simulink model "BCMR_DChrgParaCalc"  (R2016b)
settings: Solver=FixedStepDiscrete  StartTime=0.0  StopTime=10  FixedStep=0.01  RelTol=1e-3  EnableMultiTasking=on
undefined symbols (not defined in the file or in its folder): BCMR_ahDChgBattNominalCapa_C, BCMR_bCurrCalSelect_C, BCMR_bCurrIncDeltaLimEna_C, BCMR_bDChrgFulChkTenEna_C, BCMR_bDChrgFulChkThreeEna_C, BCMR_cntCoolDFC_CW, BCMR_cntSoh_CW, BCMR_G1E0PlatformSwPara_C, BCMR_iCurrDcr_C, BCMR_iDcChrgCurrAbnorm_T, BCMR_iDcChrgCurrAbnormMAP_T, BCMR_iDcChrgCurrNew_T, BCMR_iDcChrgCurrNewMAP_T, BCMR_iDcChrgCurrOld_T, BCMR_iDcChrgCurrOldAbnorm_T, BCMR_iDcChrgCurrOldAbnormMAP_T, BCMR_iDcChrgCurrOldMAP_T, BCMR_iDCCurrDecStep_C, BCMR_iDCCurrDecThrd_C, BCMR_iDCCurrDeltaLim_C, BCMR_iDCCurrDiff_C, BCMR_iDCCurrFil_C, BCMR_iDCCurrIncStep_C, BCMR_iDCCurrIncThrd_C, BCMR_iDChrgCurrCutOff_C, BCMR_kmAcmDist_C, BCMR_numCcsPwrSelc_C, BCMR_numCellVoltFull_C, BCMR_numCellVoltFullThree_C, BCMR_numCurrCalcEna, BCMR_pCcsPwrSelc_C, BCMR_pctBmsPwrRdc_C, BCMR_rCurrDcr_C, BCMR_rCurrIcr_C, BCMR_rDchrgLoadCoef_C, BCMR_tBattTempMaxFil_C, BCMR_tBattTempSelcLmtDwn_C, BCMR_tBattTempSelcLmtUp_C, BCMR_tDcChrgCellTemp1_A, BCMR_tDcChrgCellTemp2_A, BCMR_tDcChrgCellTemp_A, BCMR_tDchrgLoadLmt_C, BCMR_tiBattTempMaxFilDly_C, BCMR_tiBattTempSwitch_C, BCMR_tiCellVoltFullCnt_C, BCMR_tiCellVoltMaxFilDly_C, BCMR_tiCurrHysTimeDelay_C, BCMR_tiDcChrgPwrCCSDebs_C, BCMR_tiDChgFullPreHold_C, BCMR_tiDChrgCurrReqCalDly_C, BCMR_tiDChrgDetParaDebs_C, BCMR_tiDChrgFullBase_C, BCMR_tiDChrgFullDebs_C, BCMR_tiDChrgFulParaDebs_C, BCMR_tiDChrgFulWait_C, BCMR_tiDChrgParaBase_C, BCMR_tiHoldOnToCurrCalcOff_C, BCMR_tTempDisMapX_A, BCMR_tTempDisMapY_A, BCMR_uBattVoltOff_C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
libraries: simulink x34
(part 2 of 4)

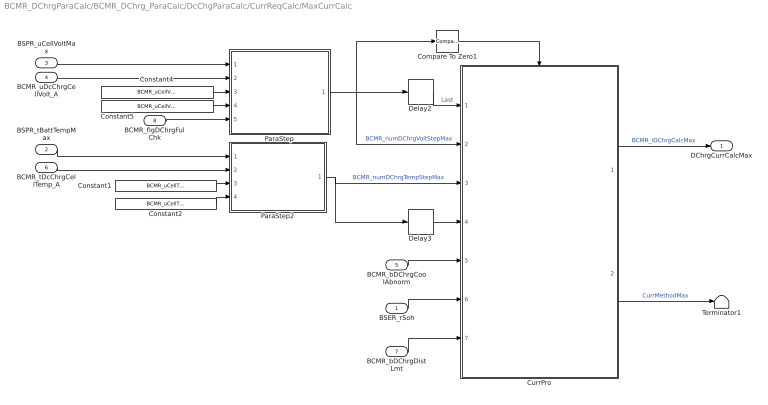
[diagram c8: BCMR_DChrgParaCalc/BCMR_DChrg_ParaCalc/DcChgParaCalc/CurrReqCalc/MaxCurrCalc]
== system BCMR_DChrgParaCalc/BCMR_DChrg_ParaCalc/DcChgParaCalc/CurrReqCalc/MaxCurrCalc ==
  BSER_rSoh : Inport
  BSPR_tBattTempMax : Inport  Port=2
  BSPR_uCellVoltMax : Inport  Port=3
  BCMR_uDcChrgCellVolt_A : Inport  Port=4
  BCMR_bDChrgCoolAbnorm : Inport  Port=5
  BCMR_tDcChrgCellTemp_A : Inport  Port=6
  BCMR_bDChrgDistLmt : Inport  Port=7
  BCMR_flgDChrgFulChk : Inport  Port=8
  Compare To Zero1 : simulink/Logic and Bit Operations/Compare To Zero  relop=>=  OutDataTypeStr=boolean
  Constant1 : Constant  Value=BCMR_uCellTempStep_A
  Constant2 : Constant  Value=BCMR_uCellTempHysRng_C
  Constant4 : Constant  Value=BCMR_uCellVoltStep_A
  Constant5 : Constant  Value=BCMR_uCellVoltHysRng_C
  CurrPro : Subsystem
  Delay2 : Delay  DelayLength=1  InitialCondition=0
  Delay3 : Delay  DelayLength=1  InitialCondition=0
  ParaStep : Stateflow chart  TreatAsAtomicUnit=on
  ParaStep2 : Stateflow chart  TreatAsAtomicUnit=on
  Terminator1 : Terminator
  DChrgCurrCalcMax : Outport
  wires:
  CurrPro/1(CurrCalc) -> DChrgCurrCalcMax/1  "BCMR_iDChrgCalcMax"
  ParaStep/1(ParaStep) -> Compare To Zero1/1, CurrPro/2(VoltStepN), Delay2/1  "BCMR_numDChrgVoltStepMax"
  Constant2/1 -> ParaStep2/4(BCMR_HysRng_C)
  ParaStep2/1(ParaStep) -> CurrPro/3(TempStepN), Delay3/1  "BCMR_numDChrgTempStepMax"
  BSPR_uCellVoltMax/1 -> ParaStep/1(BattTemp)
  BCMR_tDcChrgCellTemp_A/1 -> ParaStep2/2(BCMR_BattPara_A)
  Compare To Zero1/1 -> CurrPro/Enable
  Delay2/1 -> CurrPro/1(VoltStepL)  "Last"
  Constant1/1 -> ParaStep2/3(BCMR_ParaStep_A)
  Delay3/1 -> CurrPro/4(TempStepL)
  BCMR_uDcChrgCellVolt_A/1 -> ParaStep/2(BCMR_BattPara_A)
  BSPR_tBattTempMax/1 -> ParaStep2/1(BattTemp)
  CurrPro/2(CurrMethod) -> Terminator1/1  "CurrMethodMax"
  Constant5/1 -> ParaStep/4(BCMR_HysRng_C)
  Constant4/1 -> ParaStep/3(BCMR_ParaStep_A)
  BCMR_flgDChrgFulChk/1 -> ParaStep/5(BCMR_flgDChrgFulChk)
  BCMR_bDChrgCoolAbnorm/1 -> CurrPro/5(BCMR_bDChrgCoolAbnorm)
  BSER_rSoh/1 -> CurrPro/6(BSER_rSoh)
  BCMR_bDChrgDistLmt/1 -> CurrPro/7(BCMR_bDChrgDistLmt)

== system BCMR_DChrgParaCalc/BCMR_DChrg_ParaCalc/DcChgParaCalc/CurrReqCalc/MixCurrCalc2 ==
  BSER_rSoh : Inport
  BSPR_tBattTempMax : Inport  Port=2
  BSPR_uCellVoltMax : Inport  Port=3
  BCMR_uDcChrgCellVolt_A : Inport  Port=4
  BCMR_bDChrgCoolAbnorm : Inport  Port=5
  BCMR_tDcChrgCellTemp_A : Inport  Port=6
  BCMR_bDChrgDistLmt : Inport  Port=7
  BCMR_flgDChrgFulChk : Inport  Port=8
  Compare To Zero1 : simulink/Logic and Bit Operations/Compare To Zero  relop=>=  OutDataTypeStr=boolean
  Constant1 : Constant  Value=BCMR_uCellTempStep_A
  Constant2 : Constant  Value=BCMR_uCellTempHysRng_C
  Constant7 : Constant  Value=BCMR_uCellVoltStep_A
  Constant8 : Constant  Value=BCMR_uCellVoltHysRng_C
  CurrPro : Subsystem
  Delay2 : Delay  DelayLength=1  InitialCondition=0
  Delay3 : Delay  DelayLength=1  InitialCondition=0
  ParaStep : Stateflow chart  TreatAsAtomicUnit=on
  ParaStep1 : Stateflow chart  TreatAsAtomicUnit=on
  Terminator1 : Terminator
  DChrgCurrCalcMix2 : Outport
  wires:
  CurrPro/1(CurrCalc) -> DChrgCurrCalcMix2/1  "BCMR_iDChrgCalcMix2"
  ParaStep/1(ParaStep) -> CurrPro/2(VoltStepN), Delay2/1, Compare To Zero1/1  "BCMR_numDChrgVoltStepMix2"
  Constant2/1 -> ParaStep1/4(BCMR_HysRng_C)
  ParaStep1/1(ParaStep) -> CurrPro/3(TempStepN), Delay3/1  "BCMR_numDChrgTempStepMix2"
  BCMR_tDcChrgCellTemp_A/1 -> ParaStep1/2(BCMR_BattPara_A)
  Compare To Zero1/1 -> CurrPro/Enable
  Delay2/1 -> CurrPro/1(VoltStepL)  "Last"
  Constant1/1 -> ParaStep1/3(BCMR_ParaStep_A)
  Delay3/1 -> CurrPro/4(TempStepL)
  CurrPro/2(CurrMethod) -> Terminator1/1  "CurrMethodMin"
  BSPR_uCellVoltMax/1 -> ParaStep/1(BattTemp)
  BCMR_uDcChrgCellVolt_A/1 -> ParaStep/2(BCMR_BattPara_A)
  Constant8/1 -> ParaStep/4(BCMR_HysRng_C)
  Constant7/1 -> ParaStep/3(BCMR_ParaStep_A)
  BCMR_flgDChrgFulChk/1 -> ParaStep/5(BCMR_flgDChrgFulChk)
  BCMR_bDChrgCoolAbnorm/1 -> CurrPro/5(BCMR_bDChrgCoolAbnorm)
  BSER_rSoh/1 -> CurrPro/6(BSER_rSoh)
  BSPR_tBattTempMax/1 -> ParaStep1/1(BattTemp)
  BCMR_bDChrgDistLmt/1 -> CurrPro/7(BCMR_bDChrgDistLmt)

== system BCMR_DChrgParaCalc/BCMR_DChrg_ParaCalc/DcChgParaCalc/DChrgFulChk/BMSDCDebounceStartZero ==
  Signal : Inport
  Hearl2Fault : Inport  Port=2
  FaultStep : Inport  Port=3
  Fault2Heal : Inport  Port=4
  HealStep : Inport  Port=5
  Compare To Zero : simulink/Logic and Bit Operations/Compare To Zero  relop===  OutDataTypeStr=boolean
  FaultProcess : Subsystem
  HealProcess : Subsystem
  Switch : Switch  Criteria=u2 ~= 0
  Unit Delay : UnitDelay  SampleTime=-1  StateName=StateName
  FaultFlag : Outport  OutDataTypeStr=boolean
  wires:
  Compare To Zero/1 -> Switch/2
  Unit Delay/1 -> Compare To Zero/1, FaultProcess/4(FaultFlagOldState), HealProcess/4(FaultFlagOldState)
  HealStep/1 -> HealProcess/3(HealStep)
  Fault2Heal/1 -> HealProcess/2(Fault2Heal)
  Signal/1 -> FaultProcess/1(Signal), HealProcess/1(Signal)
  FaultStep/1 -> FaultProcess/3(FaultStep)
  Hearl2Fault/1 -> FaultProcess/2(Hearl2Fault)
  Switch/1 -> Unit Delay/1, FaultFlag/1
  HealProcess/1(FaultFlag) -> Switch/3
  FaultProcess/1(FaultFlag) -> Switch/1

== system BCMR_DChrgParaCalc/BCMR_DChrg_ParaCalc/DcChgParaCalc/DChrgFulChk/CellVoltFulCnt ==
  En : Inport
  Rst : Inport  Port=2
  Compare To Constant : simulink/Logic and Bit Operations/Compare To Constant  relop=>=  const=BCMR_numCellVoltFull_C  OutDataTypeStr=boolean
  Compare To Constant1 : simulink/Logic and Bit Operations/Compare To Constant  relop=>=  const=BCMR_numCellVoltFullThree_C  OutDataTypeStr=boolean
  Constant1 : Constant  Value=0  OutDataTypeStr=uint8
  Constant2 : Constant  OutDataTypeStr=uint8
  EdgeRising : Subsystem  TreatAsAtomicUnit=on  RTWFcnName=EdgeRising  RTWFileName=SrvLib
  EdgeRising1 : Subsystem  TreatAsAtomicUnit=on  RTWFcnName=EdgeRising  RTWFileName=SrvLib
  Timer : Subsystem
  Ten : Outport
  Three : Outport  Port=2
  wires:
  Compare To Constant/1 -> Ten/1  "BCMR_bCellVoltFullCnt"
  EdgeRising/1(y) -> Timer/1(En)
  Constant1/1 -> Timer/4(Vst)
  EdgeRising1/1(y) -> Timer/3(Rst)
  En/1 -> EdgeRising/1(u)
  Constant2/1 -> Timer/2(Cnt)
  Timer/1(Number) -> Compare To Constant1/1, Compare To Constant/1  "BCMR_numCellVoltFullCnt"
  Rst/1 -> EdgeRising1/1(u)
  Compare To Constant1/1 -> Three/1  "BCMR_bCellVoltFullTriger"

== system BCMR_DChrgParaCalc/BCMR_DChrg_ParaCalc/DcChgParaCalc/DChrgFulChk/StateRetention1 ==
  u : Inport
  clc : Inport  Port=2
  Constant1 : Constant  Value=BCMR_tiDChrgParaBase_C
  Constant2 : Constant  Value=BCMR_tiCellVoltFullCnt_C
  Constant8 : Constant  Value=single(0)
  Delay2 : Delay  DelayLength=1  InitialCondition=0
  EdgeRising : Subsystem  TreatAsAtomicUnit=on  RTWFcnName=EdgeRising  RTWFileName=SrvLib
  Logical Operator : Logic  Operator=OR  AllPortsSameDT=off  OutDataTypeStr=boolean
  Relational Operator2 : RelationalOperator  Operator=>  OutDataTypeStr=boolean  RndMeth=Simplest
  Subsystem3 : Subsystem
  Timer : Subsystem
  BCMR_bCellVoltFullTmr : Outport
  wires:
  Subsystem3/1(Q) -> Timer/1(En)  "BCMR_bCellVoltFullTmrRaw"
  Delay2/1 -> EdgeRising/1(u), Logical Operator/2
  Constant2/1 -> Relational Operator2/2
  Constant8/1 -> Timer/4(Vst)
  Timer/1(Timer) -> Relational Operator2/1
  EdgeRising/1(y) -> Timer/3(Rst)
  Constant1/1 -> Timer/2(Ts)
  Relational Operator2/1 -> BCMR_bCellVoltFullTmr/1, Delay2/1  "BCMR_bCellVoltFullTmr"
  u/1 -> Subsystem3/1(set)
  Logical Operator/1 -> Subsystem3/2(clear)
  clc/1 -> Logical Operator/1

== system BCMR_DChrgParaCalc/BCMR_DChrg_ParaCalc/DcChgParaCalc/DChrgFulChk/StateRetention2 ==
  u : Inport
  Constant4 : Constant  Value=BCMR_tiDChrgParaBase_C
  Constant5 : Constant  Value=BCMR_tiDChgFullPreHold_C
  Constant8 : Constant  Value=single(0)
  Delay2 : Delay  DelayLength=1  InitialCondition=0
  EdgeRising : Subsystem  TreatAsAtomicUnit=on  RTWFcnName=EdgeRising  RTWFileName=SrvLib
  Relational Operator2 : RelationalOperator  Operator=>  OutDataTypeStr=boolean  RndMeth=Simplest
  Subsystem3 : Subsystem
  Timer : Subsystem
  BCMR_flgDChrgFulChk : Outport
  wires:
  Subsystem3/1(Q) -> BCMR_flgDChrgFulChk/1, Timer/1(En)  "BCMR_flgDChrgFulChk"
  Delay2/1 -> EdgeRising/1(u), Subsystem3/2(clear)
  Constant5/1 -> Relational Operator2/2
  Constant8/1 -> Timer/4(Vst)
  Timer/1(Timer) -> Relational Operator2/1
  EdgeRising/1(y) -> Timer/3(Rst)
  Constant4/1 -> Timer/2(Ts)
  Relational Operator2/1 -> Delay2/1
  u/1 -> Subsystem3/1(set)  "BCMR_flgDChrgFulChkRaw"

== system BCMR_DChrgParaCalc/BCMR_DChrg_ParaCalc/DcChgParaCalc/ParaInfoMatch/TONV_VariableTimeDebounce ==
  note: Turn On Delay Time Deboune
  u : Inport
  T : Inport  Port=2
  dT : Inport  Port=3
  Add : Sum
  Constant1 : Constant  Value=0  OutDataTypeStr=single
  Constant2 : Constant  OutDataTypeStr=uint8
  Constant3 : Constant  Value=0  OutDataTypeStr=uint8
  Delay : Delay  DelayLength=1  InitialCondition=0
  MinMax : MinMax  Inputs=2
  Product : Product  OutMin=[0]  OutMax=[65535]  OutDataTypeStr=single
  Relational Operator : RelationalOperator  Operator=>  OutDataTypeStr=boolean  RndMeth=Simplest
  Switch : Switch  Criteria=u2 ~= 0
  Switch1 : Switch  Criteria=u2 ~= 0
  y : Outport
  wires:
  Switch1/1 -> Product/1
  Constant3/1 -> Switch1/3
  Constant2/1 -> Switch1/1
  u/1 -> Switch1/2, Switch/2
  dT/1 -> Switch/1
  Constant1/1 -> Switch/3
  Add/1 -> Product/2
  Product/1 -> Relational Operator/1, Delay/1
  Switch/1 -> Add/1
  Delay/1 -> MinMax/2
  Relational Operator/1 -> y/1
  T/1 -> MinMax/1, Relational Operator/2
  MinMax/1 -> Add/2

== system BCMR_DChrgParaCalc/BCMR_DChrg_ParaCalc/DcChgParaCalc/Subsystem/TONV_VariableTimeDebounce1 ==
  note: Turn On Delay Time Deboune
  u : Inport
  T : Inport  Port=2
  dT : Inport  Port=3
  Add : Sum
  Constant1 : Constant  Value=0  OutDataTypeStr=single
  Constant2 : Constant  OutDataTypeStr=uint8
  Constant3 : Constant  Value=0  OutDataTypeStr=uint8
  Delay : Delay  DelayLength=1  InitialCondition=0
  MinMax : MinMax  Inputs=2
  Product : Product  OutMin=[0]  OutMax=[65535]  OutDataTypeStr=single
  Relational Operator : RelationalOperator  Operator=>  OutDataTypeStr=boolean  RndMeth=Simplest
  Switch : Switch  Criteria=u2 ~= 0
  Switch1 : Switch  Criteria=u2 ~= 0
  y : Outport
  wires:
  Switch1/1 -> Product/1
  Constant3/1 -> Switch1/3
  Constant2/1 -> Switch1/1
  u/1 -> Switch1/2, Switch/2
  dT/1 -> Switch/1
  Constant1/1 -> Switch/3
  Add/1 -> Product/2
  Product/1 -> Relational Operator/1, Delay/1
  Switch/1 -> Add/1
  Delay/1 -> MinMax/2
  Relational Operator/1 -> y/1
  T/1 -> MinMax/1, Relational Operator/2
  MinMax/1 -> Add/2

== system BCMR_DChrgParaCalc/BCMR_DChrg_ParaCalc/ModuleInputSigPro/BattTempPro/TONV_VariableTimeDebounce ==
  note: Turn On Delay Time Deboune
  u : Inport
  T : Inport  Port=2
  dT : Inport  Port=3
  Add : Sum
  Constant1 : Constant  Value=0  OutDataTypeStr=single
  Constant2 : Constant  OutDataTypeStr=uint8
  Constant3 : Constant  Value=0  OutDataTypeStr=uint8
  Delay : Delay  DelayLength=1  InitialCondition=0
  MinMax : MinMax  Inputs=2
  Product : Product  OutMin=[0]  OutMax=[65535]  OutDataTypeStr=single
  Relational Operator : RelationalOperator  Operator=>  OutDataTypeStr=boolean  RndMeth=Simplest
  Switch : Switch  Criteria=u2 ~= 0
  Switch1 : Switch  Criteria=u2 ~= 0
  y : Outport
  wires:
  Switch1/1 -> Product/1
  Constant3/1 -> Switch1/3
  Constant2/1 -> Switch1/1
  u/1 -> Switch1/2, Switch/2
  dT/1 -> Switch/1
  Constant1/1 -> Switch/3
  Add/1 -> Product/2
  Product/1 -> Relational Operator/1, Delay/1
  Switch/1 -> Add/1
  Delay/1 -> MinMax/2
  Relational Operator/1 -> y/1
  T/1 -> MinMax/1, Relational Operator/2
  MinMax/1 -> Add/2

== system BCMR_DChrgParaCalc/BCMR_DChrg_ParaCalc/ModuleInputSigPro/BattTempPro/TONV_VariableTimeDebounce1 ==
  note: Turn On Delay Time Deboune
  u : Inport
  T : Inport  Port=2
  dT : Inport  Port=3
  Add : Sum
  Constant1 : Constant  Value=0  OutDataTypeStr=single
  Constant2 : Constant  OutDataTypeStr=uint8
  Constant3 : Constant  Value=0  OutDataTypeStr=uint8
  Delay : Delay  DelayLength=1  InitialCondition=0
  MinMax : MinMax  Inputs=2
  Product : Product  OutMin=[0]  OutMax=[65535]  OutDataTypeStr=single
  Relational Operator : RelationalOperator  Operator=>  OutDataTypeStr=boolean  RndMeth=Simplest
  Switch : Switch  Criteria=u2 ~= 0
  Switch1 : Switch  Criteria=u2 ~= 0
  y : Outport
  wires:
  Switch1/1 -> Product/1
  Constant3/1 -> Switch1/3
  Constant2/1 -> Switch1/1
  u/1 -> Switch1/2, Switch/2
  dT/1 -> Switch/1
  Constant1/1 -> Switch/3
  Add/1 -> Product/2
  Product/1 -> Relational Operator/1, Delay/1
  Switch/1 -> Add/1
  Delay/1 -> MinMax/2
  Relational Operator/1 -> y/1
  T/1 -> MinMax/1, Relational Operator/2
  MinMax/1 -> Add/2

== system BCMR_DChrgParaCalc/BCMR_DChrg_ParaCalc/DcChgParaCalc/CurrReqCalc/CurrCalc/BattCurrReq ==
  Curr : Inport
  BCMR_flgDChrgPwrRdc : Inport  Port=2
  CurrPro : Subsystem
  BCMR_iDChrgBattCurrReqCalc : Outport  OutputWhenDisabled=reset  InitialOutput=[0]
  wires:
  BCMR_flgDChrgPwrRdc/1 -> CurrPro/2(BCMR_flgDChrgPwrRdc)
  CurrPro/1(BCMR_iDChrgBattCurrReqCalc) -> BCMR_iDChrgBattCurrReqCalc/1
  Curr/1 -> CurrPro/1(CurrPro)

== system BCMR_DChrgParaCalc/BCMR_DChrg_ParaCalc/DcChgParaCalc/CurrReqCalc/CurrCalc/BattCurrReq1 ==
  CurrReq : Inport
  COMR_iDcChrgMaxCurrOutputPmtdCml : Inport  Port=2
  COMR_tiDcChrgTimeActualCcs : Inport  Port=3
  COMR_iDcChrgOutputCurrCcs : Inport  Port=4
  COMR_iDcChrgMinCurrOutputPmtdCml : Inport  Port=5
  BSPR_uPackVolt : Inport  Port=6
  BCMR_stDChrgMode : Inport  Port=7
  CurrPro : Subsystem
  BCMR_iDChrgBattCurrReqCalc : Outport  OutputWhenDisabled=reset  InitialOutput=[0]
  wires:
  COMR_iDcChrgMaxCurrOutputPmtdCml/1 -> CurrPro/2(COMR_iDcChrgMaxCurrOutputPmtdCml)
  CurrPro/1(BCMR_iDChrgBattCurrReqCalc) -> BCMR_iDChrgBattCurrReqCalc/1
  CurrReq/1 -> CurrPro/1(CurrReq)
  COMR_tiDcChrgTimeActualCcs/1 -> CurrPro/4(COMR_tiDcChrgTimeActualCcs)
  COMR_iDcChrgOutputCurrCcs/1 -> CurrPro/5(COMR_iDcChrgOutputCurrCcs)
  COMR_iDcChrgMinCurrOutputPmtdCml/1 -> CurrPro/3(COMR_iDcChrgMinCurrOutputPmtdCml)
  BSPR_uPackVolt/1 -> CurrPro/6(BSPR_uPackVolt)
  BCMR_stDChrgMode/1 -> CurrPro/7(BCMR_stDChrgMode)

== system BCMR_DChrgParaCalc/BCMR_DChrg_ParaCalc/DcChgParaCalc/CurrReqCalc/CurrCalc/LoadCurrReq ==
  COMR_pwrChrgLdReq : Inport
  BSPR_uPackVolt : Inport  Port=2
  BSPR_tBattTempMin : Inport  Port=3
  Compare To Constant : simulink/Logic and Bit Operations/Compare To Constant  relop=>=  const=BCMR_tDchrgLoadLmt_C  OutDataTypeStr=boolean
  Constant : Constant  Value=408  OutDataTypeStr=single
  Constant2 : Constant  Value=0  OutDataTypeStr=single
  Divide : Product  Inputs=*/
  Gain : Gain  Gain=1000
  Gain1 : Gain  Gain=BCMR_rDchrgLoadCoef_C
  SIgFil1 : Subsystem
  Switch : Switch  Criteria=u2 > Threshold
  Switch1 : Switch  Criteria=u2 > Threshold
  BCMR_iDChrgLoadCurrReqCalc : Outport
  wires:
  COMR_pwrChrgLdReq/1 -> Gain/1
  BSPR_uPackVolt/1 -> Switch/1, Switch/2
  Switch/1 -> Divide/2
  Constant/1 -> Switch/3
  Divide/1 -> Gain1/1
  Gain1/1 -> BCMR_iDChrgLoadCurrReqCalc/1
  BSPR_tBattTempMin/1 -> Compare To Constant/1
  Compare To Constant/1 -> Switch1/2
  Gain/1 -> [COMR_pwrChrgLdReq]
  [COMR_pwrChrgLdReq] -> SIgFil1/1(u)
  SIgFil1/1(y) -> Switch1/1
  Constant2/1 -> Switch1/3
  Switch1/1 -> Divide/1

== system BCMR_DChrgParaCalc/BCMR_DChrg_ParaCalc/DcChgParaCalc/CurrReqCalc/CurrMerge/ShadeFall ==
  In1 : Inport
  In2 : Inport  Port=2
  Add1 : Sum  Inputs=+-
  Constant3 : Constant  Value=BCMR_iCurrDcr_C  OutDataTypeStr=single
  MinMax1 : MinMax  Inputs=2
  MinMax2 : MinMax  Inputs=2
  MinMax3 : MinMax  Function=max  Inputs=2
  Relational Operator2 : RelationalOperator  OutDataTypeStr=boolean  RndMeth=Simplest
  Switch1 : Switch  Criteria=u2 > Threshold
  Unit Delay4 : UnitDelay  InitialCondition=1000  SampleTime=-1
  val : Outport
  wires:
  Constant3/1 -> Add1/2
  Add1/1 -> Switch1/1, Relational Operator2/1
  Relational Operator2/1 -> Switch1/2  "equalFlg"
  Switch1/1 -> Unit Delay4/1, val/1
  In1/1 -> MinMax1/1, MinMax3/1
  In2/1 -> MinMax1/2, MinMax3/2
  MinMax1/1 -> Switch1/3, Relational Operator2/2
  MinMax3/1 -> MinMax2/2
  Unit Delay4/1 -> MinMax2/1
  MinMax2/1 -> Add1/1

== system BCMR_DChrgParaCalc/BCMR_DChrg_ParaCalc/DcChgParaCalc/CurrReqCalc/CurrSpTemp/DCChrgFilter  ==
  In1 : Inport
  In2 : Inport  Port=2
  Abs : Abs
  Compare To Constant : simulink/Logic and Bit Operations/Compare To Constant  relop=>=  const=BCMR_iDCCurrDiff_C  OutDataTypeStr=boolean
  Subtract1 : Sum  Inputs=+-
  Switch2 : Switch  Criteria=u2 ~= 0
  Out1 : Outport
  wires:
  In2/1 -> Switch2/3, Subtract1/2
  Subtract1/1 -> Abs/1
  Abs/1 -> Compare To Constant/1
  Compare To Constant/1 -> Switch2/2
  Switch2/1 -> Out1/1
  In1/1 -> Subtract1/1, Switch2/1

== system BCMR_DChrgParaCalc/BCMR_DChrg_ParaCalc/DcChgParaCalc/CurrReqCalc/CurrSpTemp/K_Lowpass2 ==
  k : Inport
  u : Inport  Port=2
  Add : Sum
  Constant2 : Constant  Value=0
  Delay : Delay  DelayLength=1  InitialCondition=1
  Product : Product
  Subtract : Sum  Inputs=+-
  Switch1 : Switch  Criteria=u2 > Threshold
  Unit Delay : UnitDelay  SampleTime=-1
  y : Outport
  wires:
  k/1 -> Product/1
  Product/1 -> Add/1
  Constant2/1 -> Delay/1
  Unit Delay/1 -> Subtract/2, Add/2
  Subtract/1 -> Product/2
  Add/1 -> Switch1/3
  Delay/1 -> Switch1/2
  Switch1/1 -> y/1, Unit Delay/1
  u/1 -> Switch1/1, Subtract/1

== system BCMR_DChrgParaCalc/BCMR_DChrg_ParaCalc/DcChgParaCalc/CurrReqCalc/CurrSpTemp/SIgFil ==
  u : Inport
  Constant4 : Constant  Value=0  OutDataTypeStr=boolean
  Delay1 : Delay  DelayLength=1  InitialCondition=0
  Filter : Subsystem
  Switch4 : Switch  Criteria=u2 ~= 0
  Unit Delay1 : UnitDelay  InitialCondition=1  SampleTime=-1
  y : Outport
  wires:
  Delay1/1 -> Filter/2(In2)
  u/1 -> Filter/1(In1), Switch4/1
  Unit Delay1/1 -> Switch4/2
  Constant4/1 -> Unit Delay1/1
  Filter/1(Out1) -> Switch4/3
  Switch4/1 -> y/1, Delay1/1

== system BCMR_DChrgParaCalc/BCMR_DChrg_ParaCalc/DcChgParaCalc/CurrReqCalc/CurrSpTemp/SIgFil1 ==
  u : Inport
  Constant4 : Constant  Value=0  OutDataTypeStr=boolean
  Delay1 : Delay  DelayLength=1  InitialCondition=0
  Filter : Subsystem
  Switch4 : Switch  Criteria=u2 ~= 0
  Unit Delay1 : UnitDelay  InitialCondition=1  SampleTime=-1
  y : Outport
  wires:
  Switch4/1 -> Delay1/1, y/1
  Filter/1(Out1) -> Switch4/3
  Constant4/1 -> Unit Delay1/1
  Unit Delay1/1 -> Switch4/2
  u/1 -> Switch4/1, Filter/1(In1)
  Delay1/1 -> Filter/2(In2)

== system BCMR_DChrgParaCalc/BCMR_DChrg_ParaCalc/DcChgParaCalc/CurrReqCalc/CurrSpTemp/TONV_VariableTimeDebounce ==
  note: Turn On Delay Time Deboune
  u : Inport
  T : Inport  Port=2
  dT : Inport  Port=3
  Add : Sum
  Constant1 : Constant  Value=0  OutDataTypeStr=single
  Constant2 : Constant  OutDataTypeStr=uint8
  Constant3 : Constant  Value=0  OutDataTypeStr=uint8
  Delay : Delay  DelayLength=1  InitialCondition=0
  MinMax : MinMax  Inputs=2
  Product : Product  OutMin=[0]  OutMax=[65535]  OutDataTypeStr=single
  Relational Operator : RelationalOperator  Operator=>  OutDataTypeStr=boolean  RndMeth=Simplest
  Switch : Switch  Criteria=u2 ~= 0
  Switch1 : Switch  Criteria=u2 ~= 0
  y : Outport
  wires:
  Switch1/1 -> Product/1
  Constant3/1 -> Switch1/3
  Constant2/1 -> Switch1/1
  u/1 -> Switch1/2, Switch/2
  dT/1 -> Switch/1
  Constant1/1 -> Switch/3
  Add/1 -> Product/2
  Product/1 -> Relational Operator/1, Delay/1
  Switch/1 -> Add/1
  Delay/1 -> MinMax/2
  Relational Operator/1 -> y/1
  T/1 -> MinMax/1, Relational Operator/2
  MinMax/1 -> Add/2

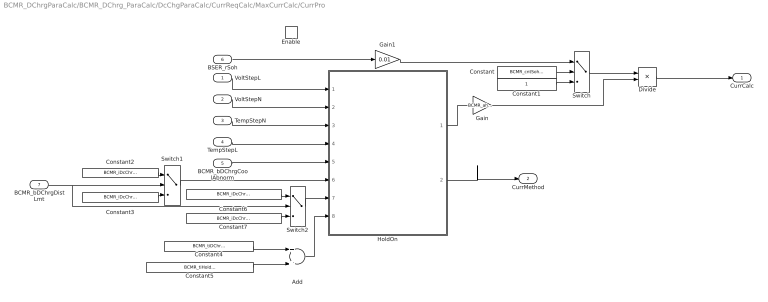
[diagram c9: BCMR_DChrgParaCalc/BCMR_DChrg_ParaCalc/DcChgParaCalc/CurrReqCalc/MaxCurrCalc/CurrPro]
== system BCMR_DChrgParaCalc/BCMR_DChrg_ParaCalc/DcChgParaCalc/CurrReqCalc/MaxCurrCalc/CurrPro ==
  VoltStepL : Inport
  VoltStepN : Inport  Port=2
  TempStepN : Inport  Port=3
  TempStepL : Inport  Port=4
  BCMR_bDChrgCoolAbnorm : Inport  Port=5
  BSER_rSoh : Inport  Port=6
  BCMR_bDChrgDistLmt : Inport  Port=7
  Enable : EnablePort  StatesWhenEnabling=reset
  Add : Sum
  Constant : Constant  Value=BCMR_cntSoh_CW
  Constant1 : Constant  OutDataTypeStr=single
  Constant2 : Constant  Value=BCMR_iDcChrgCurrOld_T
  Constant3 : Constant  Value=BCMR_iDcChrgCurrNew_T
  Constant4 : Constant  Value=BCMR_tiDChrgFulParaDebs_C
  Constant5 : Constant  Value=BCMR_tiHoldOnToCurrCalcOff_C
  Constant6 : Constant  Value=BCMR_iDcChrgCurrOldAbnorm_T
  Constant7 : Constant  Value=BCMR_iDcChrgCurrAbnorm_T
  Divide : Product  Inputs=**
  Gain : Gain  Gain=BCMR_ahDChgBattNominalCapa_C
  Gain1 : Gain  Gain=0.01  OutDataTypeStr=single
  HoldOn : Stateflow chart  TreatAsAtomicUnit=on
  Switch : Switch  Criteria=u2 > Threshold  Threshold=7
  Switch1 : Switch  Criteria=u2 > Threshold  Threshold=7
  Switch2 : Switch  Criteria=u2 > Threshold  Threshold=7
  CurrCalc : Outport  OutputWhenDisabled=reset  InitialOutput=[0]
  CurrMethod : Outport  Port=2  OutputWhenDisabled=reset  InitialOutput=[0]
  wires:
  HoldOn/1(CurrCalc) -> Gain/1
  VoltStepL/1 -> HoldOn/1(VoltStepLast)
  VoltStepN/1 -> HoldOn/2(VoltStepNext)
  TempStepN/1 -> HoldOn/3(TempStep)
  TempStepL/1 -> HoldOn/4(TempStepL)
  HoldOn/2(CurrMethod) -> CurrMethod/1
  Gain/1 -> Divide/2
  BCMR_bDChrgCoolAbnorm/1 -> HoldOn/5(BCMR_bDChrgCoolAbnorm)
  BSER_rSoh/1 -> Gain1/1
  Constant/1 -> Switch/2
  Constant1/1 -> Switch/3
  Gain1/1 -> Switch/1
  Switch/1 -> Divide/1
  Divide/1 -> CurrCalc/1
  Constant2/1 -> Switch1/1
  Constant3/1 -> Switch1/3
  Switch1/1 -> HoldOn/6(BCMR_iDcChrgCurrNew_T)
  BCMR_bDChrgDistLmt/1 -> Switch2/2, Switch1/2
  Constant6/1 -> Switch2/1
  Switch2/1 -> HoldOn/7(BCMR_iDcChrgCurrAbnorm_T)
  Constant7/1 -> Switch2/3
  Constant4/1 -> Add/1
  Constant5/1 -> Add/2
  Add/1 -> HoldOn/8(BCMR_tiHoldOnToCurrCalc_C)

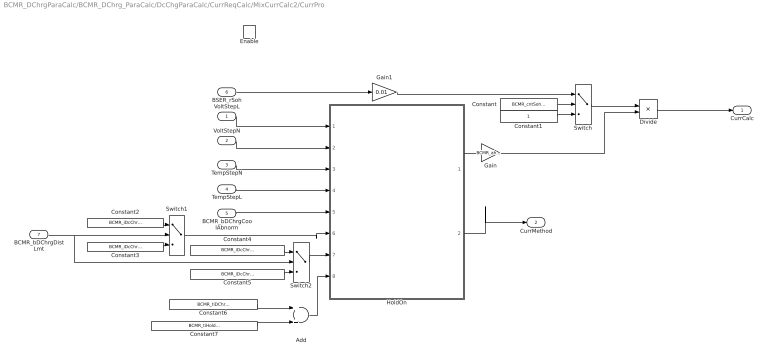
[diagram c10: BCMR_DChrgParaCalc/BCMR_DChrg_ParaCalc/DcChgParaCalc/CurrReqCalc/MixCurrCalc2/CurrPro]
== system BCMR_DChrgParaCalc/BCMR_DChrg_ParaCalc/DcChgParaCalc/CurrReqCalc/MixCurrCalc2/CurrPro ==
  VoltStepL : Inport
  VoltStepN : Inport  Port=2
  TempStepN : Inport  Port=3
  TempStepL : Inport  Port=4
  BCMR_bDChrgCoolAbnorm : Inport  Port=5
  BSER_rSoh : Inport  Port=6
  BCMR_bDChrgDistLmt : Inport  Port=7
  Enable : EnablePort  StatesWhenEnabling=reset
  Add : Sum
  Constant : Constant  Value=BCMR_cntSoh_CW
  Constant1 : Constant  OutDataTypeStr=single
  Constant2 : Constant  Value=BCMR_iDcChrgCurrOld_T
  Constant3 : Constant  Value=BCMR_iDcChrgCurrNew_T
  Constant4 : Constant  Value=BCMR_iDcChrgCurrOldAbnorm_T
  Constant5 : Constant  Value=BCMR_iDcChrgCurrAbnorm_T
  Constant6 : Constant  Value=BCMR_tiDChrgFulParaDebs_C
  Constant7 : Constant  Value=BCMR_tiHoldOnToCurrCalcOff_C
  Divide : Product  Inputs=**
  Gain : Gain  Gain=BCMR_ahDChgBattNominalCapa_C
  Gain1 : Gain  Gain=0.01  OutDataTypeStr=single
  HoldOn : Stateflow chart  TreatAsAtomicUnit=on
  Switch : Switch  Criteria=u2 > Threshold  Threshold=7
  Switch1 : Switch  Criteria=u2 > Threshold  Threshold=7
  Switch2 : Switch  Criteria=u2 > Threshold  Threshold=7
  CurrCalc : Outport  OutputWhenDisabled=reset  InitialOutput=[0]
  CurrMethod : Outport  Port=2  OutputWhenDisabled=reset  InitialOutput=[0]
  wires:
  HoldOn/1(CurrCalc) -> Gain/1
  VoltStepL/1 -> HoldOn/1(VoltStepLast)
  VoltStepN/1 -> HoldOn/2(VoltStepNext)
  TempStepN/1 -> HoldOn/3(TempStep)
  TempStepL/1 -> HoldOn/4(TempStepL)
  HoldOn/2(CurrMethod) -> CurrMethod/1
  Gain/1 -> Divide/2
  BCMR_bDChrgCoolAbnorm/1 -> HoldOn/5(BCMR_bDChrgCoolAbnorm)
  BSER_rSoh/1 -> Gain1/1
  Constant/1 -> Switch/2
  Constant1/1 -> Switch/3
  Gain1/1 -> Switch/1
  Switch/1 -> Divide/1
  Divide/1 -> CurrCalc/1
  Constant2/1 -> Switch1/1
  Constant3/1 -> Switch1/3
  Switch1/1 -> HoldOn/6(BCMR_iDcChrgCurrNew_T)
  BCMR_bDChrgDistLmt/1 -> Switch2/2, Switch1/2
  Constant4/1 -> Switch2/1
  Constant5/1 -> Switch2/3
  Switch2/1 -> HoldOn/7(BCMR_iDcChrgCurrAbnorm_T)
  Constant6/1 -> Add/1
  Add/1 -> HoldOn/8(BCMR_tiHoldOnToCurrCalc_C)
  Constant7/1 -> Add/2

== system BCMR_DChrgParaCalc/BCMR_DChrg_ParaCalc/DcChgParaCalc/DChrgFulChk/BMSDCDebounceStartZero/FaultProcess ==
  Signal : Inport
  Hearl2Fault : Inport  Port=2
  FaultStep : Inport  Port=3
  FaultFlagOldState : Inport  Port=4
  Constant : Constant  OutDataTypeStr=Inherit: Inherit via back propagation
  Constant1 : Constant  Value=0  OutDataTypeStr=Inherit: Inherit via back propagation
  Decrease : Subsystem
  Increase : Subsystem
  Relational Operator : RelationalOperator  Operator=>  OutDataTypeStr=boolean
  Switch : Switch  Criteria=u2 ~= 0
  Switch1 : Switch  Criteria=u2 ~= 0
  Switch2 : Switch  Criteria=u2 ~= 0
  Unit Delay : UnitDelay  SampleTime=-1  StateName=StateName
  Unit Delay1 : UnitDelay  SampleTime=-1  StateName=StateName
  FaultFlag : Outport
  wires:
  Unit Delay1/1 -> Switch2/2
  Unit Delay/1 -> Switch2/3
  Switch2/1 -> Increase/2(Counter), Decrease/2(Counter)
  Constant1/1 -> Switch2/1
  Constant/1 -> Switch/1
  FaultFlagOldState/1 -> Switch/3
  Switch/1 -> FaultFlag/1
  Relational Operator/1 -> Switch/2, Unit Delay1/1
  FaultStep/1 -> Increase/1(FaultStep), Decrease/1(FaultStep)
  Hearl2Fault/1 -> Relational Operator/2
  Switch1/1 -> Relational Operator/1, Unit Delay/1
  Decrease/1(FaultCnt) -> Switch1/3
  Increase/1(FaultCnt) -> Switch1/1
  Signal/1 -> Switch1/2

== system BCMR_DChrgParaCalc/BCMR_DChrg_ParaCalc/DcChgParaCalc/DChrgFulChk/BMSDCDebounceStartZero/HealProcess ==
  Signal : Inport
  Fault2Heal : Inport  Port=2
  HealStep : Inport  Port=3
  FaultFlagOldState : Inport  Port=4
  Compare To Zero : simulink/Logic and Bit Operations/Compare To Zero  relop===  OutDataTypeStr=boolean
  Constant : Constant  Value=0  OutDataTypeStr=Inherit: Inherit via back propagation
  Constant1 : Constant  Value=0  OutDataTypeStr=Inherit: Inherit via back propagation
  Decrease : Subsystem
  Increase : Subsystem
  Relational Operator : RelationalOperator  Operator=>  OutDataTypeStr=boolean
  Switch : Switch  Criteria=u2 ~= 0
  Switch1 : Switch  Criteria=u2 ~= 0
  Switch2 : Switch  Criteria=u2 ~= 0
  Unit Delay1 : UnitDelay  SampleTime=-1  StateName=StateName
  Unit Delay2 : UnitDelay  SampleTime=-1  StateName=StateName
  FaultFlag : Outport
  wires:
  Switch2/1 -> Decrease/2(Counter), Increase/2(Counter)
  Unit Delay2/1 -> Switch2/2
  Unit Delay1/1 -> Switch2/3
  Constant1/1 -> Switch2/1
  Compare To Zero/1 -> Switch1/2
  Constant/1 -> Switch/1
  FaultFlagOldState/1 -> Switch/3
  Switch/1 -> FaultFlag/1
  Relational Operator/1 -> Switch/2, Unit Delay2/1
  Signal/1 -> Compare To Zero/1
  Increase/1(HealCnt) -> Switch1/1
  Decrease/1(HealCnt) -> Switch1/3
  Switch1/1 -> Relational Operator/1, Unit Delay1/1
  Fault2Heal/1 -> Relational Operator/2
  HealStep/1 -> Increase/1(HealStep), Decrease/1(HealStep)

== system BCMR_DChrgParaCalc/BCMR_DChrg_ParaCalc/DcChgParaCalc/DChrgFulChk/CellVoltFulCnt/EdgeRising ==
  u : Inport
  Delay1 : Delay  DelayLength=1  InitialCondition=1
  Logical Operator3 : Logic  Operator=NOT  AllPortsSameDT=off  OutDataTypeStr=boolean
  Logical Operator4 : Logic  AllPortsSameDT=off  OutDataTypeStr=boolean
  y : Outport
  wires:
  Logical Operator4/1 -> y/1
  Logical Operator3/1 -> Logical Operator4/1
  u/1 -> Delay1/1, Logical Operator4/2
  Delay1/1 -> Logical Operator3/1

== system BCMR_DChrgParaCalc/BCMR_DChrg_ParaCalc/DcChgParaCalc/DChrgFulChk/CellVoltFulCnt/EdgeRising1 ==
  u : Inport
  Delay1 : Delay  DelayLength=1  InitialCondition=1
  Logical Operator3 : Logic  Operator=NOT  AllPortsSameDT=off  OutDataTypeStr=boolean
  Logical Operator4 : Logic  AllPortsSameDT=off  OutDataTypeStr=boolean
  y : Outport
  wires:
  Logical Operator4/1 -> y/1
  Logical Operator3/1 -> Logical Operator4/1
  u/1 -> Delay1/1, Logical Operator4/2
  Delay1/1 -> Logical Operator3/1

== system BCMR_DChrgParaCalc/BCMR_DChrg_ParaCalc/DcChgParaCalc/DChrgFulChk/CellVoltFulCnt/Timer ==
  En : Inport
  Cnt : Inport  Port=2
  Rst : Inport  Port=3
  Vst : Inport  Port=4
  Add : Sum
  Constant5 : Constant  Value=0  OutDataTypeStr=uint8
  Switch1 : Switch  Criteria=u2 ~= 0
  Switch2 : Switch  Criteria=u2 ~= 0
  Unit Delay : UnitDelay  SampleTime=-1
  Number : Outport
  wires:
  Unit Delay/1 -> Add/2
  Rst/1 -> Switch1/2
  En/1 -> Switch2/2
  Cnt/1 -> Switch2/1
  Constant5/1 -> Switch2/3
  Switch2/1 -> Add/1
  Vst/1 -> Switch1/1
  Switch1/1 -> Number/1, Unit Delay/1
  Add/1 -> Switch1/3

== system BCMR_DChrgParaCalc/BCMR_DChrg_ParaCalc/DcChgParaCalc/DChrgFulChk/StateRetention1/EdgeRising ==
  u : Inport
  Delay1 : Delay  DelayLength=1  InitialCondition=1
  Logical Operator3 : Logic  Operator=NOT  AllPortsSameDT=off  OutDataTypeStr=boolean
  Logical Operator4 : Logic  AllPortsSameDT=off  OutDataTypeStr=boolean
  y : Outport
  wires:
  Delay1/1 -> Logical Operator3/1
  u/1 -> Logical Operator4/2, Delay1/1
  Logical Operator3/1 -> Logical Operator4/1
  Logical Operator4/1 -> y/1

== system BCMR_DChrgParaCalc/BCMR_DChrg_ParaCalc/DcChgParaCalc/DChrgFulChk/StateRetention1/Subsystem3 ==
  set : Inport
  clear : Inport  Port=2
  Delay : Delay  DelayLength=1  InitialCondition=0
  Logical Operator : Logic  Operator=OR  AllPortsSameDT=off  OutDataTypeStr=boolean
  Logical Operator4 : Logic  AllPortsSameDT=off  OutDataTypeStr=boolean
  Logical Operator5 : Logic  Operator=NOT  AllPortsSameDT=off  OutDataTypeStr=boolean
  Q : Outport
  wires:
  Delay/1 -> Logical Operator/1
  Logical Operator4/1 -> Q/1, Delay/1
  Logical Operator/1 -> Logical Operator4/1
  Logical Operator5/1 -> Logical Operator4/2
  clear/1 -> Logical Operator5/1
  set/1 -> Logical Operator/2

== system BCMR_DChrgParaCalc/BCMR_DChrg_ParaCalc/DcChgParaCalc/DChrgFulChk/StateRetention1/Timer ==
  En : Inport
  Ts : Inport  Port=2
  Rst : Inport  Port=3
  Vst : Inport  Port=4
  Add : Sum
  Constant5 : Constant  Value=single(0)  OutDataTypeStr=single
  Switch1 : Switch  Criteria=u2 ~= 0
  Switch2 : Switch  Criteria=u2 ~= 0
  Unit Delay : UnitDelay  SampleTime=-1
  Timer : Outport
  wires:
  Unit Delay/1 -> Add/2
  Rst/1 -> Switch1/2
  En/1 -> Switch2/2
  Ts/1 -> Switch2/1
  Constant5/1 -> Switch2/3
  Switch2/1 -> Add/1
  Vst/1 -> Switch1/1
  Switch1/1 -> Timer/1, Unit Delay/1
  Add/1 -> Switch1/3

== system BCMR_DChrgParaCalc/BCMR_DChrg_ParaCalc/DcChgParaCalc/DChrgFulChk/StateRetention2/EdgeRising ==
  u : Inport
  Delay1 : Delay  DelayLength=1  InitialCondition=1
  Logical Operator3 : Logic  Operator=NOT  AllPortsSameDT=off  OutDataTypeStr=boolean
  Logical Operator4 : Logic  AllPortsSameDT=off  OutDataTypeStr=boolean
  y : Outport
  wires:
  Delay1/1 -> Logical Operator3/1
  u/1 -> Logical Operator4/2, Delay1/1
  Logical Operator3/1 -> Logical Operator4/1
  Logical Operator4/1 -> y/1

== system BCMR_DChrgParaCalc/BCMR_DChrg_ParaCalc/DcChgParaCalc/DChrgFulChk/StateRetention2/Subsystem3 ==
  set : Inport
  clear : Inport  Port=2
  Delay : Delay  DelayLength=1  InitialCondition=0
  Logical Operator : Logic  Operator=OR  AllPortsSameDT=off  OutDataTypeStr=boolean
  Logical Operator4 : Logic  AllPortsSameDT=off  OutDataTypeStr=boolean
  Logical Operator5 : Logic  Operator=NOT  AllPortsSameDT=off  OutDataTypeStr=boolean
  Q : Outport
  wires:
  Delay/1 -> Logical Operator/1
  Logical Operator4/1 -> Q/1, Delay/1
  Logical Operator/1 -> Logical Operator4/1
  Logical Operator5/1 -> Logical Operator4/2
  clear/1 -> Logical Operator5/1
  set/1 -> Logical Operator/2

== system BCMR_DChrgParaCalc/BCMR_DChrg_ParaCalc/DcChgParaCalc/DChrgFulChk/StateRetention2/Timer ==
  En : Inport
  Ts : Inport  Port=2
  Rst : Inport  Port=3
  Vst : Inport  Port=4
  Add : Sum
  Constant5 : Constant  Value=single(0)  OutDataTypeStr=single
  Switch1 : Switch  Criteria=u2 ~= 0
  Switch2 : Switch  Criteria=u2 ~= 0
  Unit Delay : UnitDelay  SampleTime=-1
  Timer : Outport
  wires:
  Unit Delay/1 -> Add/2
  Rst/1 -> Switch1/2
  En/1 -> Switch2/2
  Ts/1 -> Switch2/1
  Constant5/1 -> Switch2/3
  Switch2/1 -> Add/1
  Vst/1 -> Switch1/1
  Switch1/1 -> Timer/1, Unit Delay/1
  Add/1 -> Switch1/3

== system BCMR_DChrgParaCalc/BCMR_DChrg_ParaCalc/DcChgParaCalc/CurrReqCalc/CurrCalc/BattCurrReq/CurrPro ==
  CurrPro : Inport
  BCMR_flgDChrgPwrRdc : Inport  Port=2
  Constant1 : Constant  Value=BCMR_pctBmsPwrRdc_C  OutDataTypeStr=single
  Data Type Conversion : DataTypeConversion
  Product : Product  OutDataTypeStr=double
  Switch : Switch  Criteria=u2 > Threshold
  BCMR_iDChrgBattCurrReqCalc : Outport
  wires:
  BCMR_flgDChrgPwrRdc/1 -> Switch/2
  Product/1 -> Data Type Conversion/1
  Data Type Conversion/1 -> Switch/1
  Constant1/1 -> Product/1
  Switch/1 -> BCMR_iDChrgBattCurrReqCalc/1
  CurrPro/1 -> Switch/3, Product/2

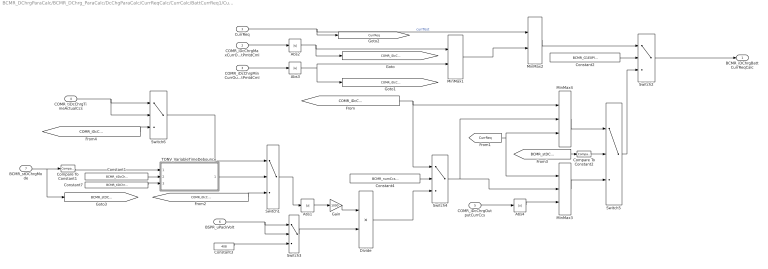
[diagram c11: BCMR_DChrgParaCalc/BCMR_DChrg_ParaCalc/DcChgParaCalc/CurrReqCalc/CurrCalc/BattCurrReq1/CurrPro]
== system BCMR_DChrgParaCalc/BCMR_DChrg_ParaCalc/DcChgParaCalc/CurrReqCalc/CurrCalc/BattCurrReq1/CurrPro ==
  CurrReq : Inport
  COMR_iDcChrgMaxCurrOutputPmtdCml : Inport  Port=2
  COMR_iDcChrgMinCurrOutputPmtdCml : Inport  Port=3
  COMR_tiDcChrgTimeActualCcs : Inport  Port=4
  COMR_iDcChrgOutputCurrCcs : Inport  Port=5
  BSPR_uPackVolt : Inport  Port=6
  BCMR_stDChrgMode : Inport  Port=7
  Abs{1..4} (4 alike) : Abs
  Compare To Constant1 : simulink/Logic and Bit Operations/Compare To Constant  relop===  const=3  OutDataTypeStr=boolean
  Compare To Constant2 : simulink/Logic and Bit Operations/Compare To Constant  relop===  const=2  OutDataTypeStr=boolean
  Constant1 : Constant  Value=BCMR_tiDcChrgPwrCCSDebs_C
  Constant2 : Constant  Value=BCMR_G1E0PlatformSwPara_C
  Constant3 : Constant  Value=408  OutDataTypeStr=single
  Constant4 : Constant  Value=BCMR_numCcsPwrSelc_C
  Constant7 : Constant  Value=BCMR_tiDChrgParaBase_C
  Divide : Product  Inputs=*/
  Gain : Gain  Gain=1000
  MinMax1 : MinMax  Function=max  Inputs=2
  MinMax2 : MinMax  Inputs=2
  MinMax3 : MinMax  Inputs=3
  MinMax4 : MinMax  Inputs=3
  Switch1 : Switch  Criteria=u2 > Threshold
  Switch2 : Switch  Criteria=u2 ~= 0
  Switch3 : Switch  Criteria=u2 > Threshold
  Switch4 : Switch  Criteria=u2 > Threshold  Threshold=2
  Switch5 : Switch  Criteria=u2 > Threshold
  Switch6 : Switch  Criteria=u2 > Threshold  Threshold=BCMR_pCcsPwrSelc_C
  TONV_VariableTimeDebounce : Subsystem  TreatAsAtomicUnit=on  RTWFcnName=TONV_VariableTimeDebounce  RTWFileName=SrvLib
  BCMR_iDChrgBattCurrReqCalc : Outport
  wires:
  CurrReq/1 -> [CurrReq], MinMax2/1  "currTest"
  COMR_iDcChrgMaxCurrOutputPmtdCml/1 -> Abs2/1
  Abs2/1 -> [COMR_iDcChrgMaxCurrOutputPmtdCmlAbs], MinMax1/1
  COMR_iDcChrgMinCurrOutputPmtdCml/1 -> Abs3/1
  Abs3/1 -> [COMR_iDcChrgMinCurrOutputPmtdCmlAbs], MinMax1/2
  MinMax1/1 -> MinMax2/2
  MinMax2/1 -> Switch2/1
  Constant2/1 -> Switch2/2
  Switch2/1 -> BCMR_iDChrgBattCurrReqCalc/1
  Switch1/1 -> Abs1/1
  Abs1/1 -> Gain/1
  Gain/1 -> Divide/1
  BSPR_uPackVolt/1 -> Switch3/2, Switch3/1
  Constant3/1 -> Switch3/3
  Switch3/1 -> Divide/2
  Divide/1 -> Switch4/3
  [COMR_iDcChrgMaxCurrOutputPmtdCmlAbs] -> Switch4/1, MinMax4/1
  [COMR_iDcChrgMinCurrOutputPmtdCmlAbs] -> Switch1/3
  Constant4/1 -> Switch4/2
  BCMR_stDChrgMode/1 -> [BCMR_stDChrgMode], Compare To Constant1/1
  COMR_iDcChrgOutputCurrCcs/1 -> Abs4/1
  Constant1/1 -> TONV_VariableTimeDebounce/2(T)
  Constant7/1 -> TONV_VariableTimeDebounce/3(dT)
  TONV_VariableTimeDebounce/1(y) -> Switch1/2
  Compare To Constant1/1 -> TONV_VariableTimeDebounce/1(u)
  [BCMR_stDChrgMode] -> Compare To Constant2/1
  Compare To Constant2/1 -> Switch5/2
  MinMax3/1 -> Switch5/3
  Switch5/1 -> Switch2/3
  MinMax4/1 -> Switch5/1
  [CurrReq] -> MinMax4/3, MinMax3/1
  Abs4/1 -> MinMax3/3
  Switch4/1 -> MinMax3/2, MinMax4/2
  COMR_tiDcChrgTimeActualCcs/1 -> Switch6/1, Switch6/2
  Switch6/1 -> Switch1/1
  [COMR_iDcChrgMinCurrOutputPmtdCmlAbs] -> Switch6/3

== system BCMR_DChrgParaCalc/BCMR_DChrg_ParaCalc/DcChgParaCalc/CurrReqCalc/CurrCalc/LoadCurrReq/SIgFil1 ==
  u : Inport
  Constant4 : Constant  Value=0  OutDataTypeStr=boolean
  Delay1 : Delay  DelayLength=1  InitialCondition=0
  Filter : Subsystem
  Switch4 : Switch  Criteria=u2 ~= 0
  Unit Delay1 : UnitDelay  InitialCondition=1  SampleTime=-1
  y : Outport
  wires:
  Delay1/1 -> Filter/2(In2)
  u/1 -> Filter/1(In1), Switch4/1
  Unit Delay1/1 -> Switch4/2
  Constant4/1 -> Unit Delay1/1
  Filter/1(Out1) -> Switch4/3
  Switch4/1 -> y/1, Delay1/1

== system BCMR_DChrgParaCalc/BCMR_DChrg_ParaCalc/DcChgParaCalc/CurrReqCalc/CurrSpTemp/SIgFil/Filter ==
  In1 : Inport
  In2 : Inport  Port=2
  Abs : Abs
  Compare To Constant : simulink/Logic and Bit Operations/Compare To Constant  relop=>=  const=BCMR_tBattTempMaxFil_C  OutDataTypeStr=boolean
  Constant5 : Constant  Value=BCMR_tiBattTempMaxFilDly_C
  Constant7 : Constant  Value=BCMR_tiDChrgParaBase_C
  Subtract1 : Sum  Inputs=+-
  Switch2 : Switch  Criteria=u2 ~= 0
  TONV_VariableTimeDebounce : Subsystem  TreatAsAtomicUnit=on  RTWFcnName=TONV_VariableTimeDebounce  RTWFileName=SrvLib
  Out1 : Outport
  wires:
  In1/1 -> Subtract1/1, Switch2/1
  Switch2/1 -> Out1/1
  Abs/1 -> Compare To Constant/1
  Subtract1/1 -> Abs/1
  In2/1 -> Subtract1/2, Switch2/3
  Constant7/1 -> TONV_VariableTimeDebounce/3(dT)
  Constant5/1 -> TONV_VariableTimeDebounce/2(T)
  TONV_VariableTimeDebounce/1(y) -> Switch2/2
  Compare To Constant/1 -> TONV_VariableTimeDebounce/1(u)

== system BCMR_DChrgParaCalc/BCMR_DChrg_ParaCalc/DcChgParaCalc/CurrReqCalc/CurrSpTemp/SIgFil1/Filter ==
  In1 : Inport
  In2 : Inport  Port=2
  Compare To Constant : simulink/Logic and Bit Operations/Compare To Constant  relop=>=  const=BCMR_uCellVoltMaxIncFil_C  OutDataTypeStr=boolean
  Compare To Constant1 : simulink/Logic and Bit Operations/Compare To Constant  relop=<=  const=BCMR_uCellVoltMaxDecFil_C  OutDataTypeStr=boolean
  Constant1 : Constant  Value=BCMR_tiCellVoltMaxFilDly_C
  Constant2 : Constant  Value=BCMR_tiDChrgParaBase_C
  Constant5 : Constant  Value=BCMR_tiCellVoltMaxFilDly_C
  Constant7 : Constant  Value=BCMR_tiDChrgParaBase_C
  Subtract1 : Sum  Inputs=+-
  Subtract2 : Sum  Inputs=+-
  Switch1 : Switch  Criteria=u2 ~= 0
  Switch2 : Switch  Criteria=u2 ~= 0
  TONV_VariableTimeDebounce : Subsystem  TreatAsAtomicUnit=on  RTWFcnName=TONV_VariableTimeDebounce  RTWFileName=SrvLib
  TONV_VariableTimeDebounce1 : Subsystem  TreatAsAtomicUnit=on  RTWFcnName=TONV_VariableTimeDebounce  RTWFileName=SrvLib
  Out1 : Outport
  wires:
  In2/1 -> Switch1/3, Subtract2/2, Subtract1/2
  Subtract1/1 -> Compare To Constant/1
  Compare To Constant/1 -> TONV_VariableTimeDebounce/1(u)
  Switch2/1 -> Out1/1
  In1/1 -> Subtract2/1, Switch1/1, Subtract1/1, Switch2/1
  Switch1/1 -> Switch2/3
  Subtract2/1 -> Compare To Constant1/1
  Constant7/1 -> TONV_VariableTimeDebounce/3(dT)
  Constant5/1 -> TONV_VariableTimeDebounce/2(T)
  TONV_VariableTimeDebounce/1(y) -> Switch2/2
  Constant2/1 -> TONV_VariableTimeDebounce1/3(dT)
  Constant1/1 -> TONV_VariableTimeDebounce1/2(T)
  TONV_VariableTimeDebounce1/1(y) -> Switch1/2
  Compare To Constant1/1 -> TONV_VariableTimeDebounce1/1(u)

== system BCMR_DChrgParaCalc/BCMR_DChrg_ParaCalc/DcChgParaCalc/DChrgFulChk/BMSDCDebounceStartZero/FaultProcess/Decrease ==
  FaultStep : Inport
  Counter : Inport  Port=2
  Constant : Constant  Value=0  OutDataTypeStr=Inherit: Inherit via back propagation
  Nomal : Subsystem
  Relational Operator : RelationalOperator  OutDataTypeStr=boolean
  Switch : Switch  Criteria=u2 ~= 0
  FaultCnt : Outport
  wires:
  Constant/1 -> Switch/3
  FaultStep/1 -> Relational Operator/2, Nomal/1(FaultStep)
  Counter/1 -> Relational Operator/1, Nomal/2(Counter)
  Switch/1 -> FaultCnt/1
  Nomal/1(FaultCnt) -> Switch/1
  Relational Operator/1 -> Switch/2

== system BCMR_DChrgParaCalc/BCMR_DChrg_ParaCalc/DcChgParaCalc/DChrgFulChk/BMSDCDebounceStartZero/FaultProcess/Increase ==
  FaultStep : Inport
  Counter : Inport  Port=2
  Add : Sum  AccumDataTypeStr=uint16  OutDataTypeStr=uint16
  Saturation : Saturate  UpperLimit=60000  LowerLimit=0
  FaultCnt : Outport
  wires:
  Saturation/1 -> FaultCnt/1
  Add/1 -> Saturation/1
  Counter/1 -> Add/2
  FaultStep/1 -> Add/1

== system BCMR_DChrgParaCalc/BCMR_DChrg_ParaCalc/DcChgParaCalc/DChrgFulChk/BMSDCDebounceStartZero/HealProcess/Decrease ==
  HealStep : Inport
  Counter : Inport  Port=2
  Constant : Constant  Value=0  OutDataTypeStr=Inherit: Inherit via back propagation
  Nomal : Subsystem
  Relational Operator : RelationalOperator  OutDataTypeStr=boolean
  Switch : Switch  Criteria=u2 ~= 0
  HealCnt : Outport
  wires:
  Constant/1 -> Switch/3
  Relational Operator/1 -> Switch/2
  Nomal/1(HealCnt) -> Switch/1
  Switch/1 -> HealCnt/1
  Counter/1 -> Relational Operator/1, Nomal/2(Counter)
  HealStep/1 -> Relational Operator/2, Nomal/1(HealStep)

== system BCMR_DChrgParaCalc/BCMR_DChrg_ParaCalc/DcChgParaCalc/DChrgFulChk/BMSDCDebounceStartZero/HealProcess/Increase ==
  HealStep : Inport
  Counter : Inport  Port=2
  Add : Sum  AccumDataTypeStr=uint16  OutDataTypeStr=uint16
  Saturation : Saturate  UpperLimit=60000  LowerLimit=0
  HealCnt : Outport
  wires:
  HealStep/1 -> Add/1
  Counter/1 -> Add/2
  Add/1 -> Saturation/1
  Saturation/1 -> HealCnt/1

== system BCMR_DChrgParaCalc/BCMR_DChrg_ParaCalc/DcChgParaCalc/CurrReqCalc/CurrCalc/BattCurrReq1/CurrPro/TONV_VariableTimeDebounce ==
  note: Turn On Delay Time Deboune
  u : Inport
  T : Inport  Port=2
  dT : Inport  Port=3
  Add : Sum
  Constant1 : Constant  Value=0  OutDataTypeStr=single
  Constant2 : Constant  OutDataTypeStr=uint8
  Constant3 : Constant  Value=0  OutDataTypeStr=uint8
  Delay : Delay  DelayLength=1  InitialCondition=0
  MinMax : MinMax  Inputs=2
  Product : Product  OutMin=[0]  OutMax=[65535]  OutDataTypeStr=single
  Relational Operator : RelationalOperator  Operator=>  OutDataTypeStr=boolean  RndMeth=Simplest
  Switch : Switch  Criteria=u2 ~= 0
  Switch1 : Switch  Criteria=u2 ~= 0
  y : Outport
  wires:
  Switch1/1 -> Product/1
  Constant3/1 -> Switch1/3
  Constant2/1 -> Switch1/1
  u/1 -> Switch1/2, Switch/2
  dT/1 -> Switch/1
  Constant1/1 -> Switch/3
  Add/1 -> Product/2
  Product/1 -> Relational Operator/1, Delay/1
  Switch/1 -> Add/1
  Delay/1 -> MinMax/2
  Relational Operator/1 -> y/1
  T/1 -> MinMax/1, Relational Operator/2
  MinMax/1 -> Add/2

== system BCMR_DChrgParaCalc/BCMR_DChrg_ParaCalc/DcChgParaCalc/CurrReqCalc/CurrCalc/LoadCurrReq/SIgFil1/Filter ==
  In1 : Inport
  In2 : Inport  Port=2
  Abs : Abs
  Compare To Constant : simulink/Logic and Bit Operations/Compare To Constant  relop=>=  const=COMR_pwrChrgLdReqFil_C  OutDataTypeStr=boolean
  Constant5 : Constant  Value=COMR_tipwrChrgLdReqFilDly_C
  Constant7 : Constant  Value=BCMR_tiDChrgParaBase_C
  Subtract1 : Sum  Inputs=+-
  Switch2 : Switch  Criteria=u2 ~= 0
  TONV_VariableTimeDebounce : Subsystem  TreatAsAtomicUnit=on  RTWFcnName=TONV_VariableTimeDebounce  RTWFileName=SrvLib
  Out1 : Outport
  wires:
  In1/1 -> Subtract1/1, Switch2/1
  Switch2/1 -> Out1/1
  Abs/1 -> Compare To Constant/1
  Subtract1/1 -> Abs/1
  In2/1 -> Switch2/3, Subtract1/2
  Constant7/1 -> TONV_VariableTimeDebounce/3(dT)
  Constant5/1 -> TONV_VariableTimeDebounce/2(T)
  Compare To Constant/1 -> TONV_VariableTimeDebounce/1(u)
  TONV_VariableTimeDebounce/1(y) -> Switch2/2

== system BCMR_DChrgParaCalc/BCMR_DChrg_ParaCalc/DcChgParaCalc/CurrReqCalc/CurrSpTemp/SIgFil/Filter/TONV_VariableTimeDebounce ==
  note: Turn On Delay Time Deboune
  u : Inport
  T : Inport  Port=2
  dT : Inport  Port=3
  Add : Sum
  Constant1 : Constant  Value=0  OutDataTypeStr=single
  Constant2 : Constant  OutDataTypeStr=uint8
  Constant3 : Constant  Value=0  OutDataTypeStr=uint8
  Delay : Delay  DelayLength=1  InitialCondition=0
  MinMax : MinMax  Inputs=2
  Product : Product  OutMin=[0]  OutMax=[65535]  OutDataTypeStr=single
  Relational Operator : RelationalOperator  Operator=>  OutDataTypeStr=boolean  RndMeth=Simplest
  Switch : Switch  Criteria=u2 ~= 0
  Switch1 : Switch  Criteria=u2 ~= 0
  y : Outport
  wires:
  Switch1/1 -> Product/1
  Constant3/1 -> Switch1/3
  Constant2/1 -> Switch1/1
  u/1 -> Switch1/2, Switch/2
  dT/1 -> Switch/1
  Constant1/1 -> Switch/3
  Add/1 -> Product/2
  Product/1 -> Relational Operator/1, Delay/1
  Switch/1 -> Add/1
  Delay/1 -> MinMax/2
  Relational Operator/1 -> y/1
  T/1 -> MinMax/1, Relational Operator/2
  MinMax/1 -> Add/2

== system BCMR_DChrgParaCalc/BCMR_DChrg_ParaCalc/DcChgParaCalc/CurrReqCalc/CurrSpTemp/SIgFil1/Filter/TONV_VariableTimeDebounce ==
  note: Turn On Delay Time Deboune
  u : Inport
  T : Inport  Port=2
  dT : Inport  Port=3
  Add : Sum
  Constant1 : Constant  Value=0  OutDataTypeStr=single
  Constant2 : Constant  OutDataTypeStr=uint8
  Constant3 : Constant  Value=0  OutDataTypeStr=uint8
  Delay : Delay  DelayLength=1  InitialCondition=0
  MinMax : MinMax  Inputs=2
  Product : Product  OutMin=[0]  OutMax=[65535]  OutDataTypeStr=single
  Relational Operator : RelationalOperator  Operator=>  OutDataTypeStr=boolean  RndMeth=Simplest
  Switch : Switch  Criteria=u2 ~= 0
  Switch1 : Switch  Criteria=u2 ~= 0
  y : Outport
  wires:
  Switch1/1 -> Product/1
  Constant3/1 -> Switch1/3
  Constant2/1 -> Switch1/1
  u/1 -> Switch1/2, Switch/2
  dT/1 -> Switch/1
  Constant1/1 -> Switch/3
  Add/1 -> Product/2
  Product/1 -> Relational Operator/1, Delay/1
  Switch/1 -> Add/1
  Delay/1 -> MinMax/2
  Relational Operator/1 -> y/1
  T/1 -> MinMax/1, Relational Operator/2
  MinMax/1 -> Add/2

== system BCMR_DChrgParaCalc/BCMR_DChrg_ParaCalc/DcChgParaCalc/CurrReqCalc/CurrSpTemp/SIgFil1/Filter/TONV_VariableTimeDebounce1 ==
  note: Turn On Delay Time Deboune
  u : Inport
  T : Inport  Port=2
  dT : Inport  Port=3
  Add : Sum
  Constant1 : Constant  Value=0  OutDataTypeStr=single
  Constant2 : Constant  OutDataTypeStr=uint8
  Constant3 : Constant  Value=0  OutDataTypeStr=uint8
  Delay : Delay  DelayLength=1  InitialCondition=0
  MinMax : MinMax  Inputs=2
  Product : Product  OutMin=[0]  OutMax=[65535]  OutDataTypeStr=single
  Relational Operator : RelationalOperator  Operator=>  OutDataTypeStr=boolean  RndMeth=Simplest
  Switch : Switch  Criteria=u2 ~= 0
  Switch1 : Switch  Criteria=u2 ~= 0
  y : Outport
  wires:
  MinMax/1 -> Add/2
  T/1 -> Relational Operator/2, MinMax/1
  Relational Operator/1 -> y/1
  Delay/1 -> MinMax/2
  Switch/1 -> Add/1
  Product/1 -> Delay/1, Relational Operator/1
  Add/1 -> Product/2
  Constant1/1 -> Switch/3
  dT/1 -> Switch/1
  u/1 -> Switch/2, Switch1/2
  Constant2/1 -> Switch1/1
  Constant3/1 -> Switch1/3
  Switch1/1 -> Product/1

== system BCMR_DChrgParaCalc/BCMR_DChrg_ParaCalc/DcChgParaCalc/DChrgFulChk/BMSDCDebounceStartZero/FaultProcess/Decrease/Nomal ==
  FaultStep : Inport
  Counter : Inport  Port=2
  Add : Sum  Inputs=+-  AccumDataTypeStr=uint16  OutDataTypeStr=uint16
  FaultCnt : Outport
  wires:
  Add/1 -> FaultCnt/1
  FaultStep/1 -> Add/2
  Counter/1 -> Add/1

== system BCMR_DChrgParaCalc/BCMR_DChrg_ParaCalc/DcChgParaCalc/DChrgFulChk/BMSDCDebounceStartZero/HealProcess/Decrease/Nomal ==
  HealStep : Inport
  Counter : Inport  Port=2
  Add : Sum  Inputs=+-  AccumDataTypeStr=uint16  OutDataTypeStr=uint16
  HealCnt : Outport
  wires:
  Counter/1 -> Add/1
  HealStep/1 -> Add/2
  Add/1 -> HealCnt/1

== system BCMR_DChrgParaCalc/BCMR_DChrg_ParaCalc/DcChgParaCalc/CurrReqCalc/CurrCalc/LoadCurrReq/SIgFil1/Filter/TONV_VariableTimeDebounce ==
  note: Turn On Delay Time Deboune
  u : Inport
  T : Inport  Port=2
  dT : Inport  Port=3
  Add : Sum
  Constant1 : Constant  Value=0  OutDataTypeStr=single
  Constant2 : Constant  OutDataTypeStr=uint8
  Constant3 : Constant  Value=0  OutDataTypeStr=uint8
  Delay : Delay  DelayLength=1  InitialCondition=0
  MinMax : MinMax  Inputs=2
  Product : Product  OutMin=[0]  OutMax=[65535]  OutDataTypeStr=single
  Relational Operator : RelationalOperator  Operator=>  OutDataTypeStr=boolean  RndMeth=Simplest
  Switch : Switch  Criteria=u2 ~= 0
  Switch1 : Switch  Criteria=u2 ~= 0
  y : Outport
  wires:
  Switch1/1 -> Product/1
  Constant3/1 -> Switch1/3
  Constant2/1 -> Switch1/1
  u/1 -> Switch1/2, Switch/2
  dT/1 -> Switch/1
  Constant1/1 -> Switch/3
  Add/1 -> Product/2
  Product/1 -> Relational Operator/1, Delay/1
  Switch/1 -> Add/1
  Delay/1 -> MinMax/2
  Relational Operator/1 -> y/1
  T/1 -> MinMax/1, Relational Operator/2
  MinMax/1 -> Add/2
